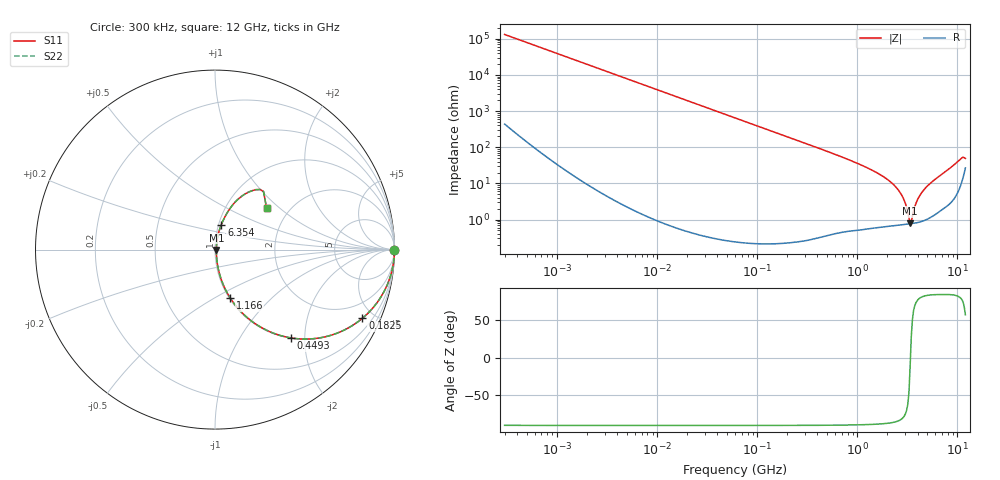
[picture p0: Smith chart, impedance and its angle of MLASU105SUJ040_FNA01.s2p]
! MLASU105SUJ040_FNA01  S-PARAMETER MODEL  ( General Type )
! Model Generated by TAIYO YUDEN Corporation (http://www.ty-top.com)
! Version 2.0
! TAIYO YUDEN Control No. 120810
! Copyright(c) 2011 TAIYO YUDEN CO.,LTD. All Rights Reserved.
! Product Description (link to TY-COMPAS)
! https://ds.yuden.co.jp/TYCOMPAS/or/detail?pn=MLASU105SUJ040CFNA01&u=M
! Products Name : Multilayer Ceramic Capacitors
! Characteristics :
!  Capacitance : 4 pF , Rated Voltage : 50V , TCC : UJ / U2J
!  Case Size : 1.0 x 0.5 / 0.039 x 0.02 [mm/inch] , Thickness : 0.5 / 0.02 [mm/inch]
!  (Conditions: Temperature = 25 degC , DC Bias Current/Voltage = 0A / 0V)
! External Node Assignments :
!  1  o---| |---o  2
! GND o---------o GND
! Frequency Range : 0.3MHz  -  12000MHz  [ 401 STEP ]
# MHz S RI R 50
! Freq[MHz].  S11 Real  S11 Imag  S21 Real  S21 Imag  S12 Real  S12 Imag  S22 Real  S22 Imag
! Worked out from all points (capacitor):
!   401 points, 300 kHz to 12 GHz, reference 50 ohm
!   read as one part in series: C = 4.05 pF near 316.3 kHz
!   lowest |Z| = 786 mohm at 3.365 GHz (marker M1)
!   series resonance near 3.392 GHz, so ESL is about 540 pH
!   S11 on the Smith chart (normalised r, x): 300 kHz: open; 182.5 MHz: 1.00, -4.29; 449.3 MHz: 1.01, -1.72; 1.166 GHz: 1.01, -0.59; 6.354 GHz: 1.03, +0.29; 12 GHz: 1.53, +0.83
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0.3  1 -0.000764  3.13e-06 0.000764  3.13e-06 0.000764  1 -0.000764
1.769972  1 -0.0045  2.26e-05 0.0045  2.26e-05 0.0045  1 -0.0045
10.44266  0.9993 -0.0266  0.000712 0.0266  0.000712 0.0266  0.9993 -0.0266
60  0.9771 -0.1493  0.0229 0.1493  0.0229 0.1493  0.9771 -0.1493
182.544  0.8214 -0.3825  0.1786 0.3825  0.1786 0.3825  0.8214 -0.3825
353.9943  0.5464 -0.4966  0.4536 0.4966  0.4536 0.4966  0.5464 -0.4966
449.3064  0.4249 -0.4924  0.5751 0.4924  0.5751 0.4924  0.4249 -0.4924
723.8279  0.2136 -0.4056  0.7864 0.4056  0.7864 0.4056  0.2136 -0.4056
1166.079  0.0852 -0.2703  0.9148 0.2703  0.9148 0.2703  0.0852 -0.2703
2088.533  0.0197 -0.1137  0.9803 0.1137  0.9803 0.1137  0.0197 -0.1137
2448.343  0.0126 -0.0753  0.9874 0.0753  0.9874 0.0753  0.0126 -0.0753
2795.104  0.00911 -0.0443  0.9909 0.0443  0.9909 0.0443  0.00911 -0.0443
3026.31  0.00802 -0.026  0.992 0.026  0.992 0.026  0.00802 -0.026
3276.641  0.00761 -0.00783  0.9924 0.00783  0.9924 0.00783  0.00761 -0.00783
3364.605  0.00761 -0.00168  0.9924 0.00168  0.9924 0.00168  0.00761 -0.00168
3547.679  0.00784 0.00934  0.9922 -0.00934  0.9922 -0.00934  0.00784 0.00934
3944.255  0.00912 0.0313  0.9909 -0.0313  0.9909 -0.0313  0.00912 0.0313
4385.161  0.0116 0.0532  0.9884 -0.0532  0.9884 -0.0532  0.0116 0.0532
6354.153  0.0352 0.1392  0.9648 -0.1392  0.9648 -0.1392  0.0352 0.1392
8503.825  0.0897 0.2378  0.9103 -0.2378  0.9103 -0.2378  0.0897 0.2378
10511.28  0.2028 0.327  0.7972 -0.327  0.7972 -0.327  0.2028 0.327
12000  0.287 0.2331  0.713 -0.2331  0.713 -0.2331  0.287 0.2331
